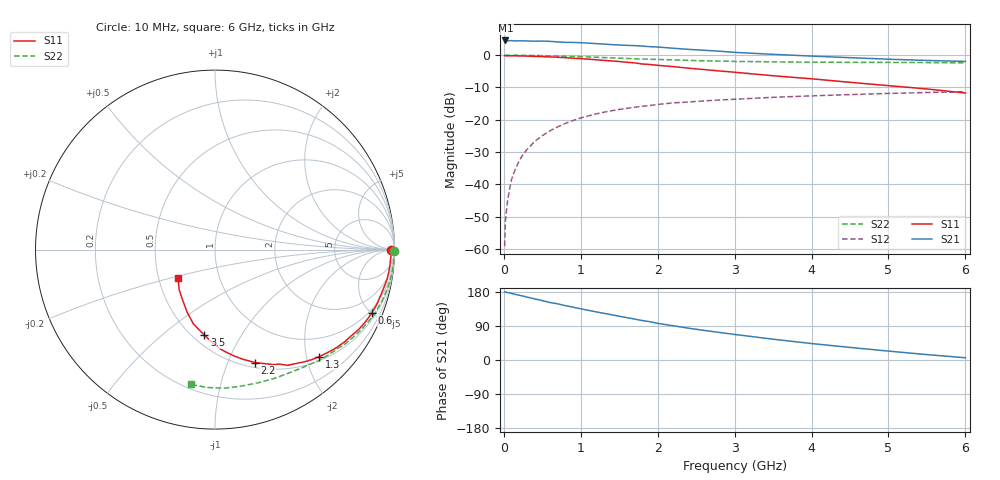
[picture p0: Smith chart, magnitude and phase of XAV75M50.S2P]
! SIEMENS Discrete & RF Semiconductors
! BFY180
! Si NPN RF Bipolar Junction Transistor in MICRO-X
! VCE = 0.75 V  IC = 0.5 mA
! Common Emitter S-Parameters:  May  1997
# GHz  S  MA  R  50
!  f  S11  S21  S12  S22
! GHz  MAG  ANG  MAG  ANG  MAG  ANG  MAG  ANG
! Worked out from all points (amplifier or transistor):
!   36 points, 10 MHz to 6 GHz, reference 50 ohm
!   highest |S21| = 4.6 dB at 20 MHz (marker M1)
!   |S21| within 3 dB of that: start of sweep to 2.573 GHz
!   unconditionally stable (mu >= 1): 4.045 GHz to end of sweep
!   at 250 MHz: K = 0.07, MSG = 17.6 dB, |S12| = -30.8 dB
!   at 1.4 GHz: K = 0.46, MSG = 10.2 dB, |S12| = -17.2 dB
!   at 6 GHz: K = 1.09, MAG = 2.9 dB, |S12| = -11.3 dB
!   S11 on the Smith chart (normalised r, x): 10 MHz: open; 600 MHz: 0.79, -5.02; 1.3 GHz: 0.58, -2.25; 2.2 GHz: 0.55, -1.25; 3.5 GHz: 0.57, -0.71; 6 GHz: 0.63, -0.21
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0.01  0.9826 -0.2  1.678 179.9  0.0011 93.4  0.9983 -0.3
0.02  0.9801 -0.7  1.694 179.2  0.0027 85.3  0.9999 -0.6
0.05  0.9816 -1.8  1.669 177.9  0.0058 86.4  0.9986 -1.3
0.1  0.9793 -3.8  1.687 175.6  0.0119 88.7  0.9947 -2.5
0.2  0.9761 -7.4  1.673 170.8  0.0232 84.7  0.9959 -5.0
0.3  0.9693 -11.0  1.665 166.1  0.0345 81.4  0.994 -7.5
0.4  0.9594 -14.6  1.651 161.4  0.0461 78.8  0.9908 -9.9
0.5  0.9521 -18.6  1.658 156.7  0.0568 75.5  0.9851 -12.4
0.6  0.9426 -22.0  1.641 151.7  0.0674 73.0  0.9794 -14.8
0.8  0.9164 -29.0  1.583 143.4  0.0877 67.4  0.9655 -19.5
1.1  0.8687 -39.1  1.54 131.1  0.1149 59.3  0.9391 -26.2
1.3  0.8326 -45.7  1.488 123.2  0.1311 54.4  0.9201 -30.5
1.7  0.7609 -57.9  1.408 108.0  0.1561 46.1  0.8811 -38.2
2  0.6971 -65.9  1.34 96.7  0.1729 40.7  0.8601 -43.5
2.2  0.6666 -70.7  1.284 90.4  0.1823 37.1  0.8471 -46.9
2.4  0.6299 -75.8  1.233 84.0  0.1887 34.1  0.831 -50.0
2.8  0.571 -84.4  1.156 72.8  0.2026 28.8  0.8112 -55.7
3.5  0.4809 -97.0  1.033 54.9  0.2229 20.9  0.79 -65.4
4  0.4313 -106.2  0.97 43.4  0.2345 15.5  0.7797 -72.2
4.5  0.3806 -114.2  0.916 33.2  0.2454 10.6  0.7747 -79.0
5.5  0.3002 -131.7  0.83 14.2  0.2645 0.9  0.7695 -93.2
6  0.2598 -142.3  0.802 5.9  0.2714 -4.0  0.7631 -100.3
